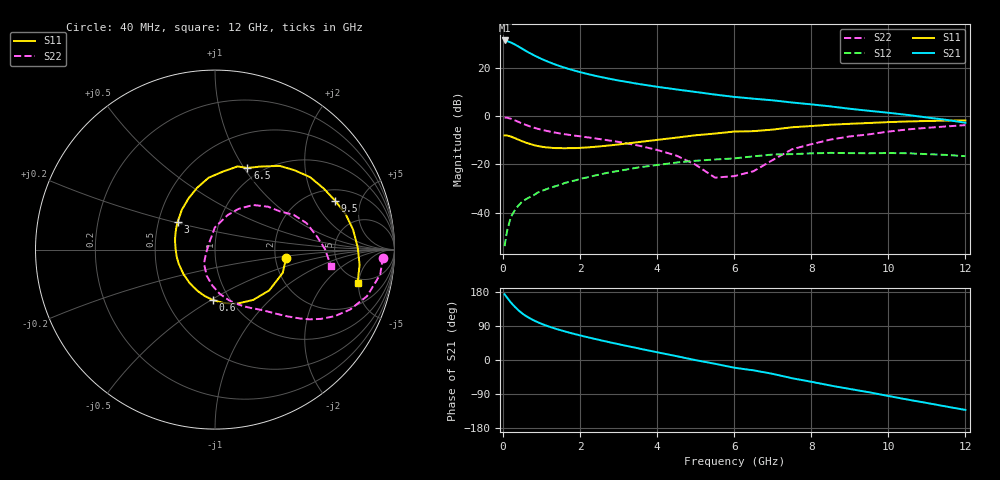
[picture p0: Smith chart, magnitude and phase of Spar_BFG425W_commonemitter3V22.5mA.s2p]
! Filename: 322bfg425.001
! BFG425W Field C1
! V1=8.513E-001V,V2=3.000E+000V, I1=2.993E-004A, I2=2.254E-002A
# GHz  S  MA  R 50
!  S11  S21  S12  S22
!Freq(GHz)  Mag  Ang  Mag  Ang  Mag  Ang  Mag  Ang
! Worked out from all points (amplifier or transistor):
!   44 points, 40 MHz to 12 GHz, reference 50 ohm
!   highest |S21| = 31.5 dB at 40 MHz (marker M1)
!   |S21| within 3 dB of that: start of sweep to 450.3 MHz
!   unconditionally stable (mu >= 1): 1.276 GHz to end of sweep
!   at 700 MHz: K = 0.78, MSG = 29.9 dB, |S12| = -33.6 dB
!   at 2.4 GHz: K = 1.15, MAG = 18.3 dB, |S12| = -24.6 dB
!   at 12 GHz: K = 1.34, MAG = 3.4 dB, |S12| = -16.6 dB
!   S11 on the Smith chart (normalised r, x): 40 MHz: 2.29, -0.26; 600 MHz: 0.83, -0.51; 3 GHz: 0.63, +0.21; 6.5 GHz: 0.87, +1.03; 9.5 GHz: 2.61, +2.97; 12 GHz: 4.33, -4.84
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0.04  0.399 -6.8  37.39 173.3  0.002 76.2  0.936 -2.7
0.1  0.399 -19.0  36.34 165.2  0.004 82.2  0.931 -8.6
0.2  0.378 -37.0  34.04 152.1  0.008 76.0  0.886 -17.0
0.3  0.352 -52.9  31.03 140.9  0.011 72.0  0.824 -23.9
0.4  0.325 -67.9  27.95 131.2  0.014 68.1  0.762 -29.2
0.5  0.301 -81.2  25.09 122.6  0.017 65.8  0.704 -33.3
0.6  0.281 -92.5  22.51 115.7  0.019 64.1  0.655 -36.4
0.7  0.265 -102.4  20.32 109.8  0.021 62.9  0.612 -38.9
0.8  0.251 -111.9  18.44 104.4  0.023 62.0  0.577 -40.9
0.9  0.24 -120.1  16.83 99.7  0.026 61.3  0.548 -42.7
1  0.233 -127.8  15.44 95.5  0.028 60.6  0.523 -44.3
1.2  0.223 -141.2  13.21 88.0  0.032 59.3  0.482 -47.3
1.6  0.216 -163.6  10.17 75.5  0.041 56.5  0.423 -52.6
2.2  0.225 170.5  7.5 60.0  0.054 50.9  0.363 -61.5
3  0.259 143.6  5.505 41.7  0.073 41.5  0.292 -74.7
4.5  0.359 106.0  3.594 10.2  0.109 19.9  0.152 -107.9
5.5  0.436 84.4  2.813 -10.0  0.126 4.2  0.053 -159.4
6.5  0.489 68.4  2.31 -27.3  0.147 -8.1  0.072 106.6
8.5  0.666 37.3  1.596 -67.5  0.173 -45.2  0.327 49.5
9.5  0.723 22.1  1.293 -85.1  0.17 -61.8  0.42 30.5
10.5  0.777 8.3  1.063 -104.5  0.17 -80.4  0.531 16.1
12  0.816 -13.2  0.732 -131.8  0.148 -110.3  0.652 -8.0
